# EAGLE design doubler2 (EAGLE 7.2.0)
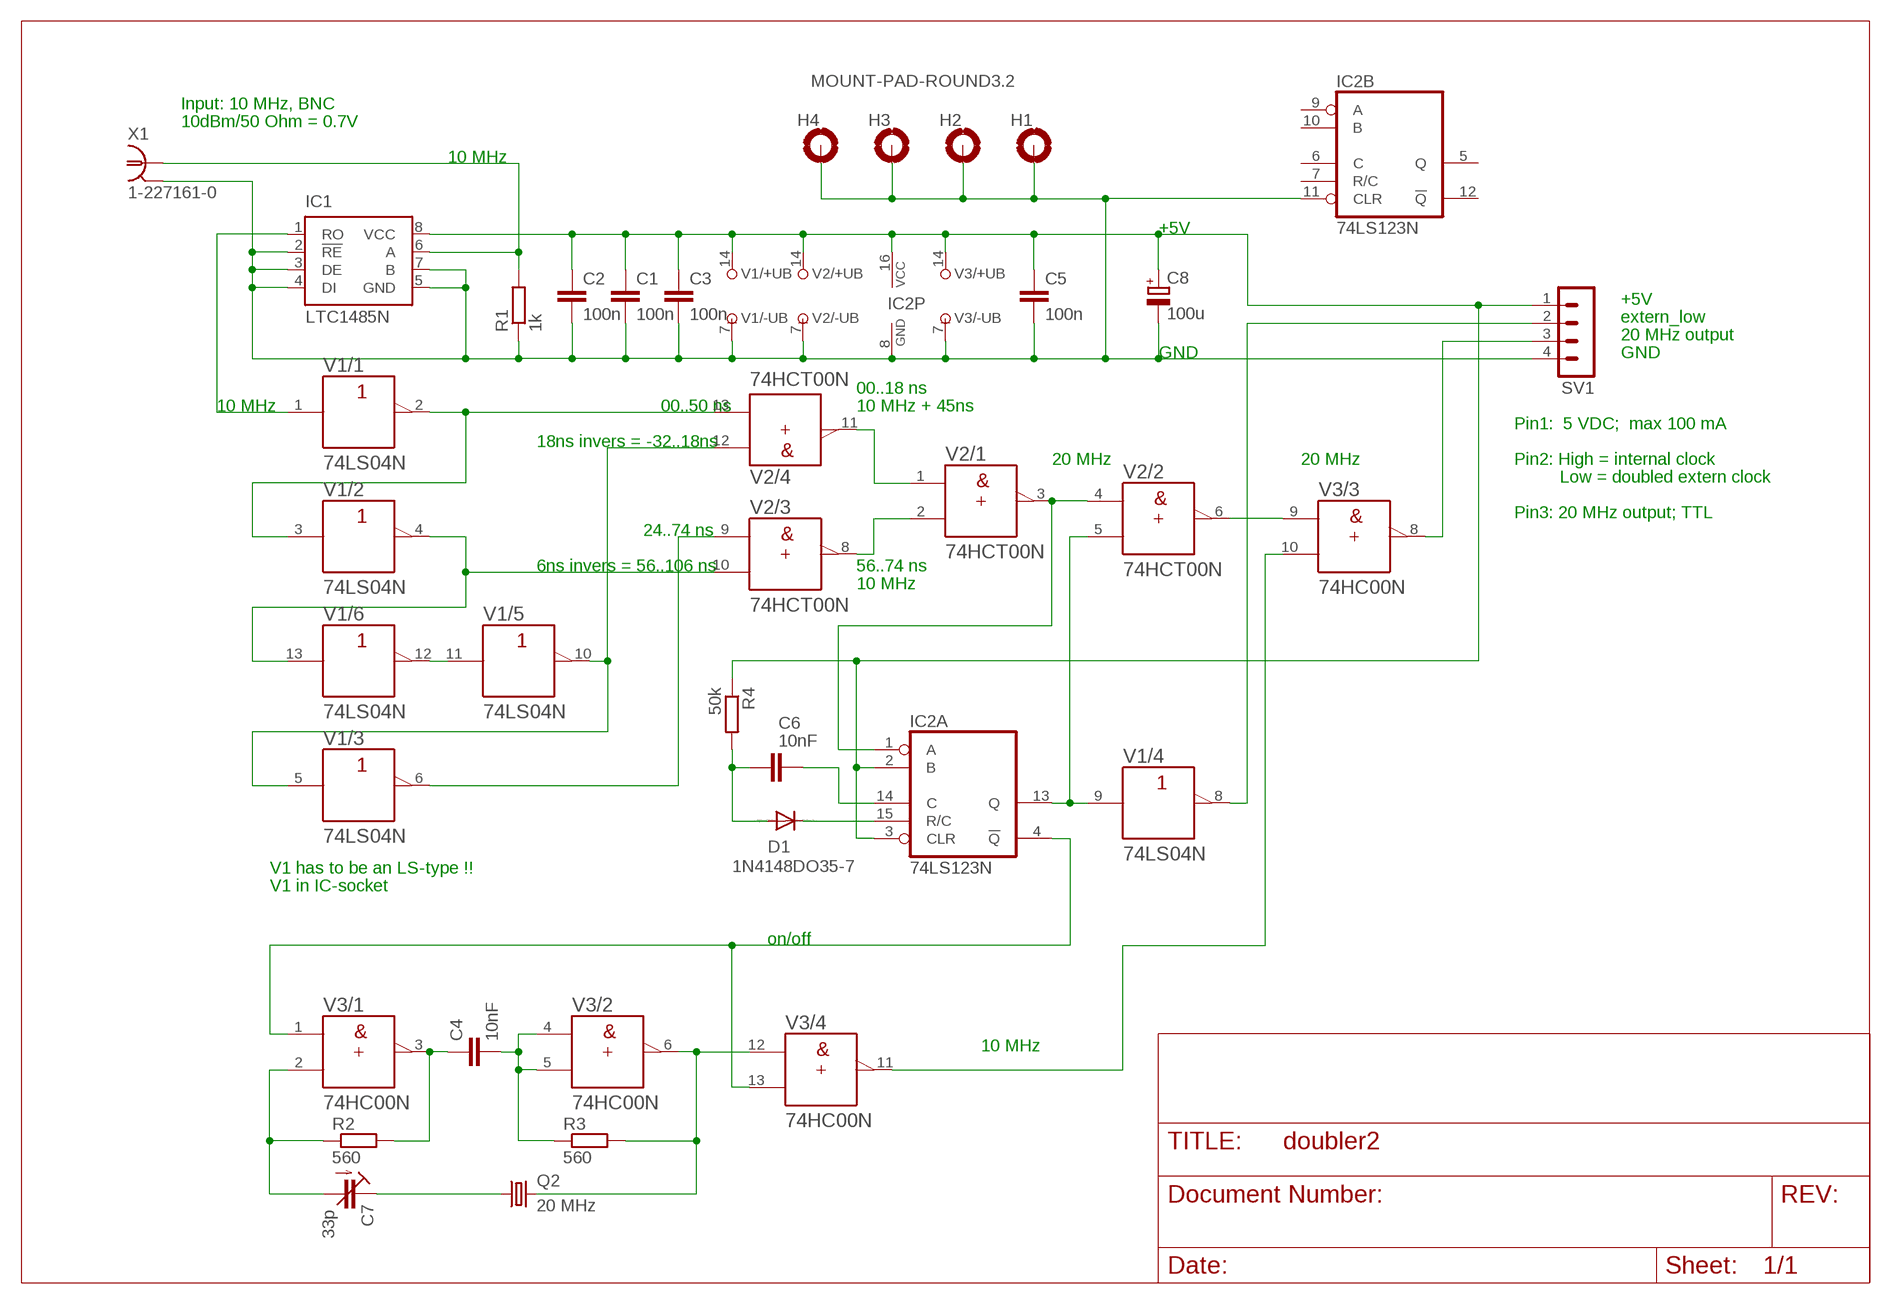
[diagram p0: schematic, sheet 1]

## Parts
C1  100n  C-EU050-025X075  [C050-025X075]
C2  100n  C-EU050-025X075  [C050-025X075]
C3  100n  C-EU050-025X075  [C050-025X075]
C4  10nF  C-EU050-025X075  [C050-025X075]
C5  100n  C-EU050-025X075  [C050-025X075]
C6  10nF  C-EU050-025X075  [C050-025X075]
C7  33p  C-TRIMM3040.427  [CTRIM3040.427]
C8  100u  CPOL-EUE5-8.5  [E5-8,5]
D1  1N4148DO35-7  [DO35-7]
H1  MOUNT-PAD-ROUND3.2  [3,2-PAD]
H2  MOUNT-PAD-ROUND3.2  [3,2-PAD]
H3  MOUNT-PAD-ROUND3.2  [3,2-PAD]
H4  MOUNT-PAD-ROUND3.2  [3,2-PAD]
IC1  LTC1485N  LTC485N  [DIL08]
IC2  74LS123N  [DIL16]
Q2  20 MHz  CRYTALHC49S  [HC49/S]
R1  1k  R-EU_0207/10  [0207/10]
R2  560  R-EU_0207/10  [0207/10]
R3  560  R-EU_0207/10  [0207/10]
R4  50k  R-EU_0207/10  [0207/10]
SV1  MA04-1  [MA04-1]
V1  74LS04N  7404N  [DIL14]
V2  74HCT00N  [DIL14]
V3  74HC00N  [DIL14]
X1  1-227161-0  [AMP_227161]

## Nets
GND: C1.2 C2.2 C3.2 C5.2 C8.- H1.B3,2(MOUNT) H2.B3,2(MOUNT) H3.B3,2(MOUNT) H4.B3,2(MOUNT) IC1.2(!RE) IC1.3(DE) IC1.4(DI) IC1.5(GND) IC1.7(B) IC2.8(P:GND) IC2.11(B:CLR) R1.1 SV1.4 V1.7(/-UB:-UB) V2.7(/-UB:-UB) V3.7(/-UB:-UB) X1.2 X1.3 X1.4
N$1: IC1.1(RO) V1.1(/1:A)
N$2: V1.6(/3:Y) V2.9(/3:A)
N$3: V2.1(/1:A) V2.11(/4:Y)
N$4: V1.2(/1:Y) V1.3(/2:A) V2.13(/4:B)
N$5: V2.2(/1:B) V2.8(/3:Y)
N$6: IC2.1(A:A) V2.3(/1:Y) V2.4(/2:A)
N$7: C7.1A(E) Q2.1
N$8: IC1.6(A) R1.2 X1.1
N$9: C4.1 R2.2 V3.3(/1:Y)
N$10: V1.4(/2:Y) V1.13(/6:A) V2.10(/3:B)
N$11: V1.11(/5:A) V1.12(/6:Y)
N$12: V1.5(/3:A) V1.10(/5:Y) V2.12(/4:A)
N$13: C4.2 R3.1 V3.4(/2:A) V3.5(/2:B)
N$14: C1.1 C2.1 C3.1 C5.1 C8.+ IC1.8(VCC) IC2.2(A:B) IC2.3(A:CLR) IC2.16(P:VCC) R4.1 SV1.1 V1.14(/+UB:+UB) V2.14(/+UB:+UB) V3.14(/+UB:+UB)
N$15: C7.2(A) R2.1 V3.2(/1:B)
N$16: SV1.3 V3.8(/3:Y)
N$17: Q2.2 R3.2 V3.6(/2:Y) V3.12(/4:A)
N$18: V3.10(/3:B) V3.11(/4:Y)
N$20: IC2.4(A:!Q) V3.1(/1:A) V3.13(/4:B)
N$21: IC2.13(A:Q) V1.9(/4:A) V2.5(/2:B)
N$22: V2.6(/2:Y) V3.9(/3:A)
N$23: SV1.2 V1.8(/4:Y)
N$24: C6.2 D1.A R4.2
N$25: C6.1 IC2.14(A:C)
N$26: D1.C IC2.15(A:R/C)
Unconnected: IC2.5(B:Q) IC2.6(B:C) IC2.7(B:R/C) IC2.9(B:A) IC2.10(B:B) IC2.12(B:!Q)

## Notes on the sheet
- Input: 10 MHz, BNC
- 10dBm/50 Ohm = 0.7V
- 10 MHz
- +5V
- +5V
- extern_low
- 20 MHz output
- GND | GND
- 00..18 ns
- 10 MHz | 00..50 ns | 10 MHz + 45ns
- Pin1:  5 VDC;  max 100 mA
- 18ns invers = -32..18ns
- 20 MHz | 20 MHz | Pin2: High = internal clock
- Low = doubled extern clock
- Pin3: 20 MHz output; TTL
- 24..74 ns
- 6ns invers = 56..106 ns | 56..74 ns
- 10 MHz
- V1 has to be an LS-type !!
- V1 in IC-socket
- on/off
- 10 MHz

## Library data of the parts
C1-C6 = rcl:C-EU: CAPACITOR, European symbol
C7 = rcl:C-TRIMM: Trimm capacitor
C8 = rcl:CPOL-EU: POLARIZED CAPACITOR, European symbol
D1 = diode:1N4148: DIODE
H1-H4 = holes:MOUNT-PAD-ROUND: MOUNTING PAD, round
IC1 = linear-technology:LTC485: Low Power RS485 Interface Transceiver Source: http://www.linear.com/pc/downloadDocument.do?navId=H0,C1,C1007,C1017,P2064,D1718; OC_FARNELL: unknown; OC_NEWARK: unknown
IC2 = 74xx-eu:74*123: Retriggerable monostable MULTIVIBRATOR
Q2 = crystal:CRYTAL: CRYSTAL
R1-R4 = rcl:R-EU_: RESISTOR, European symbol
SV1 = con-lstb:MA04-1: PIN HEADER; OC_FARNELL: unknown; OC_NEWARK: unknown
V1 = 74ttl-din:74*04: Hex INVERTER
V2 V3 = 74ttl-din:74*00: Quad 2-input NAND gate
X1 = sprut1:?227161*: JACK, RIGHT ANGLE, 50 OHM, PCB, BNC; MF: TYCO ELECTRONICS; MPN: 1-227161; OC_FARNELL: unknown; OC_NEWARK: 33B3200

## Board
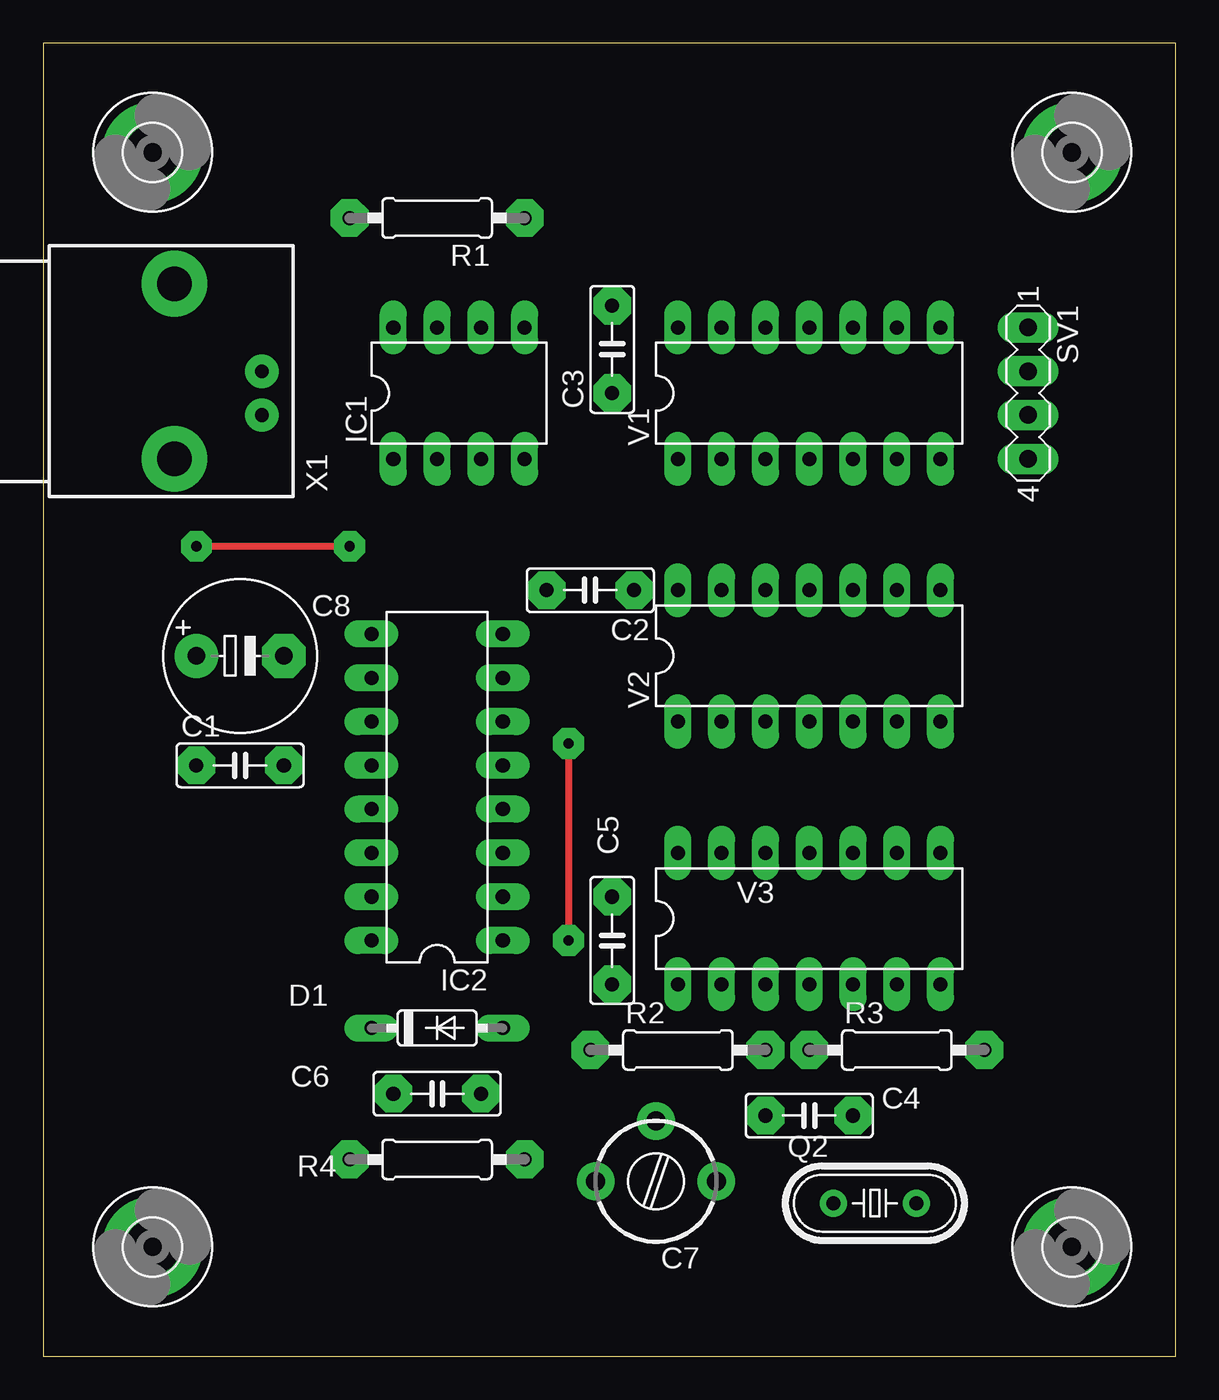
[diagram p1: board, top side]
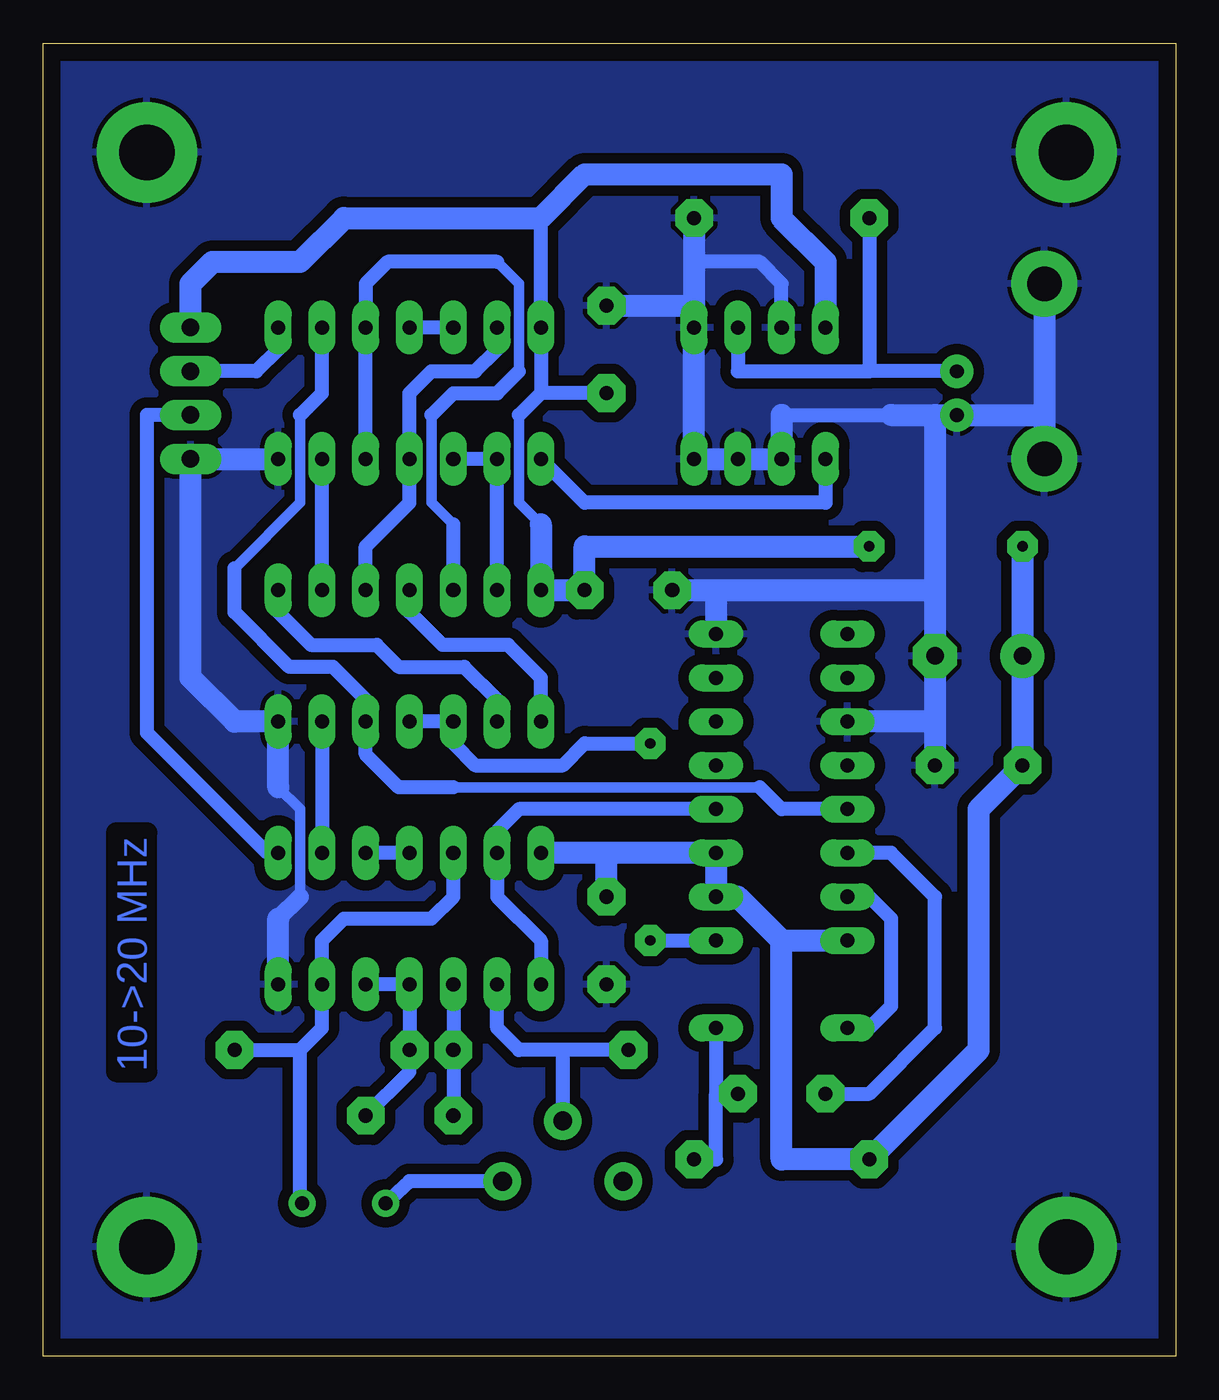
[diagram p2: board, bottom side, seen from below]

Size 65.71 x 76.19 mm. Coordinates in mm from the lower left corner, seen from the top.
Outline: 0,0 65.71,0 65.71,76.19 0,76.19 0,0
Copper layers (1*16): Top 0.035mm / dielectric 1.5mm / Bottom 0.035mm
Design rules "default *": minimum track width 10mil, minimum drill 24mil, track to track 8mil, track to pad 8mil, pad to pad 8mil, via to via 8mil, smd to smd 8mil, copper to edge 40mil, drill to drill 8mil, minimum pad ring 15mil, minimum via ring 8mil, stop-mask expansion 4mil, vias tented up to drill 0mil, thermal gap 10mil

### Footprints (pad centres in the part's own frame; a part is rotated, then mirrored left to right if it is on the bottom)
C050-025X075 = drill 0.813 pad 2.184 octagon: 1 -2.54,0; 2 2.54,0
CTRIM3040.427 = drill 1.1 pad 2.184: 1A -3.5,0; 1B 3.5,0; 2 0,-3.5
E5-8,5 = drill 1.016 pad 2.54: + -2.54,0 | drill 1.016 pad 2.54 octagon: - 2.54,0
DO35-7 = drill 0.813 long: A 3.81,0; C -3.81,0
3,2-PAD = drill 3.2 pad 5.842: B3,2 0,0
DIL08 = drill 0.813 long: 1 -3.81,-3.81; 2 -1.27,-3.81; 3 1.27,-3.81; 4 3.81,-3.81; 5 3.81,3.81; 6 1.27,3.81; 7 -1.27,3.81; 8 -3.81,3.81
DIL16 = drill 0.813 long: 1 -8.89,-3.81; 2 -6.35,-3.81; 3 -3.81,-3.81; 4 -1.27,-3.81; 5 1.27,-3.81; 6 3.81,-3.81; 7 6.35,-3.81; 8 8.89,-3.81; 9 8.89,3.81; 10 6.35,3.81; 11 3.81,3.81; 12 1.27,3.81; 13 -1.27,3.81; 14 -3.81,3.81; 15 -6.35,3.81; 16 -8.89,3.81
HC49/S = drill 0.813: 1 -2.413,0; 2 2.413,0
0207/10 = drill 0.813 pad 2.184 octagon: 1 -5.08,0; 2 5.08,0
MA04-1 = drill 1.016 long: 1 -3.81,0; 2 -1.27,0; 3 1.27,0; 4 3.81,0
DIL14 = drill 0.813 long: 1 -7.62,-3.81; 2 -5.08,-3.81; 3 -2.54,-3.81; 4 0,-3.81; 5 2.54,-3.81; 6 5.08,-3.81; 7 7.62,-3.81; 8 7.62,3.81; 9 5.08,3.81; 10 2.54,3.81; 11 0,3.81; 12 -2.54,3.81; 13 -5.08,3.81; 14 -7.62,3.81
AMP_227161 = drill 0.8 pad 1.93: 1 0,-5.08; 2 -2.54,-5.08 | drill 2 pad 3.81: 3 -5.08,0; 4 5.08,0

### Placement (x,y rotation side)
C1  11.43,34.29 0 top
C2  31.75,44.45 180 top
C3  33.02,58.42 90 top
C4  44.45,13.97 0 top
C5  33.02,24.13 270 top
C6  22.86,15.24 0 top
C7  35.56,10.16 180 top
C8  11.43,40.64 0 top
D1  22.86,19.05 0 top
H1  59.69,69.85 0 top
H2  6.35,69.85 0 top
H3  6.35,6.35 0 top
H4  59.69,6.35 0 top
IC1  24.13,55.88 0 top
IC2  22.86,33.02 90 top
Q2  48.26,8.89 0 top
R1  22.86,66.04 180 top
R2  36.83,17.78 0 top
R3  49.53,17.78 0 top
R4  22.86,11.43 0 top
SV1  57.15,55.88 270 top
V1  44.45,55.88 0 top
V2  44.45,40.64 0 top
V3  44.45,25.4 0 top
X1  7.62,57.15 90 top

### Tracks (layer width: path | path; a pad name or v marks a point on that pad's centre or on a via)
GND
  Bottom 0.406: 22.86,54.61 13.97,54.61
  Bottom 0.61: 50.8,26.67 50.8,31.75 52.07,33.02
  Bottom 0.813: IC1.7 22.86,62.23 24.13,63.5 27.94,63.5 | 22.86,54.61 16.51,54.61
  Bottom 1.016: 52.07,25.4 50.8,26.67
  Bottom 1.27: R1.1 27.94,63.5 IC1.5 | IC1.5 IC1.4 IC1.3 IC1.2 22.86,54.61 | 16.51,54.61 13.97,54.61 | 13.97,54.61 X1.2 7.62,54.61 | V1.7 SV1.4 57.15,39.37 54.61,36.83 V2.7 52.07,33.02 | V3.7 52.07,25.4 | X1.4 7.62,54.61 | 7.62,54.61 X1.3 | 13.97,36.83 IC2.11 | C3.2 27.94,60.96 IC1.5 | IC2.8 26.67,44.45 C2.2 13.97,44.45 | 13.97,36.83 C8.- 13.97,44.45 | 13.97,36.83 C1.2 | 13.97,54.61 13.97,44.45
  pour Bottom (isolate 0.61): 0,76.2 66.04,76.2 66.04,0 0,0
N$1
  Bottom 0.813: IC1.1 20.32,49.53 34.29,49.53 V1.1
N$2
  Bottom 0.813: V2.9 V1.6
N$3
  Bottom 0.813: V2.1 36.83,39.37 38.73,41.27 42.55,41.27 44.45,43.18 V2.11
N$4
  Bottom 0.813: V2.13 V1.2 V1.3
N$5
  Bottom 0.813: V2.8 52.07,43.18 50.16,41.27 46.35,41.27 45.09,40.01 41.27,40.01 39.37,38.1 V2.2
N$6  (via drill 0.6 pad 1.78)
  Top 0.406: v30.48,35.56 v30.48,24.13
  Bottom 0.813: V2.4 V2.3 41.91,35.56 40.64,34.29 35.56,34.29 34.29,35.56 v30.48,35.56 | v30.48,24.13 IC2.1
N$7
  Bottom 0.813: C7.1A 44.45,10.16 Q2.1
N$8
  Bottom 0.813: 17.78,57.15 25.4,57.15 IC1.6 | R1.2 17.78,57.15 | X1.1 17.78,57.15
N$9
  Bottom 0.813: V3.3 R2.2 C4.1
N$10
  Bottom 0.813: V1.13 39.37,58.42 40.64,57.15 43.18,57.15 44.45,55.88 V1.4 44.45,49.53 46.99,46.99 V2.10
N$11
  Bottom 0.813: V1.12 V1.11
N$12
  Bottom 0.61: 41.91,48.26 43.18,49.53 43.18,54.61 | 38.1,57.15 38.1,62.23 39.37,63.5
  Bottom 0.813: V1.5 V1.10 46.99,62.23 45.72,63.5 39.37,63.5 | V2.12 41.91,48.26 | 43.18,54.61 41.91,55.88 39.37,55.88 38.1,57.15
N$13
  Bottom 0.813: V3.5 V3.4 R3.1 44.45,16.51 C4.2
N$14  (via drill 0.6 pad 1.78)
  Top 0.406: v17.78,46.99 v8.89,46.99
  Bottom 0.61: 38.1,54.61 38.1,49.53 36.83,48.26
  Bottom 0.813: 36.83,55.88 V1.14 36.83,66.04 | 36.83,55.88 38.1,54.61 | C3.1 36.83,55.88
  Bottom 1.27: 36.83,48.26 V2.14 C2.1 34.29,46.99 v17.78,46.99 | IC1.8 20.32,63.5 22.86,66.04 22.86,68.58 34.29,68.58 36.83,66.04 48.26,66.04 50.8,63.5 55.88,63.5 57.15,62.23 SV1.1 | 22.86,24.13 25.4,26.67 IC2.2 IC2.3 33.02,29.21 | 22.86,24.13 IC2.16 | 22.86,24.13 22.86,11.43 R4.1 11.43,17.78 11.43,31.75 C1.1 C8.+ v8.89,46.99 | 33.02,29.21 V3.14 | C5.1 33.02,29.21
N$15
  Bottom 0.813: R2.1 35.56,17.78 | 35.56,17.78 38.1,17.78 39.37,19.05 V3.2 | C7.2 35.56,17.78
N$16
  Bottom 0.813: V3.8 52.7,29.21 59.69,36.2 59.69,54.61 SV1.3
N$17
  Bottom 0.406: Q2.2 50.8,8.89
  Bottom 0.813: R3.2 50.8,17.78 | 50.8,17.78 49.53,19.05 V3.6 49.53,24.13 48.26,25.4 43.18,25.4 41.91,26.67 V3.12 | 50.8,8.89 50.8,17.78
N$18
  Bottom 0.813: V3.11 V3.10
N$20
  Bottom 0.61: 39.37,30.48 V3.13
  Bottom 0.813: V3.13 39.37,26.67 36.83,24.13 V3.1 | IC2.4 38.1,31.75 39.37,30.48
N$21
  Bottom 0.61: 54.61,45.72 50.8,49.53 50.8,54.61 | 24.13,33.02 41.91,33.02
  Bottom 0.813: 54.61,45.72 54.61,43.18 51.44,40.01 48.9,40.01 46.99,38.1 V2.5 46.99,34.93 45.09,33.02 41.91,33.02 | 50.8,54.61 49.53,55.88 V1.9 | IC2.13 22.86,31.75 24.13,33.02
N$22
  Bottom 0.813: V2.6 V3.9
N$23
  Bottom 0.813: V1.8 52.07,58.42 53.34,57.15 SV1.2
N$24
  Bottom 0.813: D1.A 26.67,15.24 | 26.67,15.24 C6.2 | R4.2 26.67,11.43 26.67,15.24
N$25
  Bottom 0.813: C6.1 17.78,15.24 13.97,19.05 13.97,26.67 16.51,29.21 IC2.14
N$26
  Bottom 0.813: IC2.15 17.78,26.67 16.51,25.4 16.51,20.32 17.78,19.05 D1.C

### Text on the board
Bottom: 10->20 MHz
